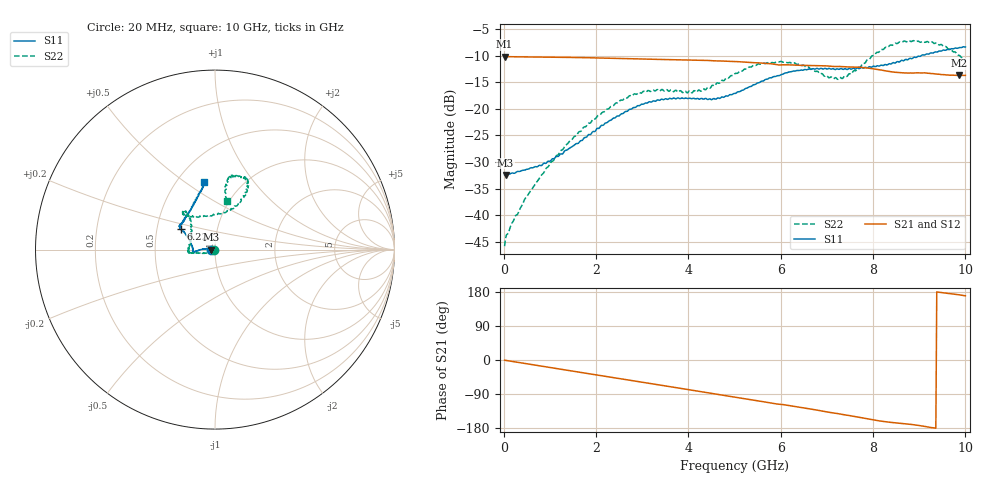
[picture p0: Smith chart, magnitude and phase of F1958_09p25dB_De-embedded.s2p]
! Integrated Device Technology
! Corporate Headquarters
! 6024 Silver Creek Valley Road
! San Jose, CA 95138  USA
! Phone:  1-408-284-8200
! Toll Free:  1-800-223-1366
! Webpage:  http://www.idt.com/
! Timing and RF Division
! 515 Groton Road, Suite 102
! Westford, MA 01886-6024
! Device:  F1958
! Description: 7-bit 0.25 dB Digital Step Attenuator
! Frequency:  0.001 -  6.000 GHz
! Package:  4x4 mm Thin QFN Plastic Package: 24 pin
! Ports:  2 RF, 12 DC
!  Pin  1  = D0
!  Pin  2  = VDD
!  Pin  3  = VMODE
!  Pin  4  = GND
!  Pin  5  = RF1  =  Port 1
!  Pin  6  = GND
!  Pin  7  = GND
!  Pin  8  = GND
!  Pin  9  = GND
!  Pin 10  = GND
!  Pin 11  = GND
!  Pin 12  = GND
!  Pin 13  = GND
!  Pin 14  = RF2  =  Port 2
!  Pin 15  = GND
!  Pin 16  = LE
!  Pin 17  = CLK
!  Pin 18  = DATA
!  Pin 19  = D6
!  Pin 20  = D5
!  Pin 21  = D4
!  Pin 22  = D3
!  Pin 23  = D2
!  Pin 24  = D1
! State:  37
! Atten State:  9.25 dB
! Voltage:  +3.30 Volts
! Current:  0.258 mA
! Data:  The device was measured on a F1958 evaluation board which has
!  individual transmission lines to the RF pins.  Data was collected
!  using a calibrated network analyzer.  The evaluation board was
!  de-embedded using Automatic Fixture Removal (AFR).
!  The reference plane is the edge of the package pin.
! Misc:
!  Action Tracker AT0419
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# GHz S dB R 50
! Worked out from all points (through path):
!   500 points, 20 MHz to 10 GHz, reference 50 ohm
!   highest |S21| = -10.19 dB at 20 MHz (marker M1); lowest = -13.7 dB at 9.86 GHz (marker M2)
!   group delay of S21, straight-line fit = 53.7 ps
!   lowest |S11| = -32.4 dB at 40 MHz (marker M3), VSWR 1.05, Z = 47.7 - j0.0687 ohm
!   |S11| at or under -10 dB: start of sweep to 9.048 GHz
!   |S22| runs from -45.8 to -7.2 dB; largest |S21 - S12| = 0.00084
!   S11 on the Smith chart (normalised r, x): 20 MHz: 0.95, -0.00; 6.22 GHz: 0.66, +0.16; 10 GHz: 0.67, +0.59
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0.02  -32.40 -178.2  -10.19 -0.5  -10.19 -0.5  -45.77 -157.7
0.04  -32.43 -178.3  -10.20 -0.9  -10.20 -0.9  -44.31 -151.7
0.22  -32.09 177.9  -10.23 -4.5  -10.23 -4.5  -40.86 -145.9
0.68  -30.84 173.9  -10.27 -13.5  -10.27 -13.4  -34.19 -144.1
1.16  -28.93 175.6  -10.31 -22.9  -10.31 -22.9  -28.71 -150.3
1.7  -25.92 176.7  -10.40 -33.3  -10.39 -33.3  -23.88 -162.4
2.58  -20.90 -176.9  -10.56 -50.5  -10.55 -50.5  -18.35 -171.0
3.36  -18.38 -171.8  -10.73 -65.7  -10.73 -65.8  -16.58 -175.4
4.22  -18.13 -175.0  -10.88 -82.4  -10.89 -82.5  -16.48 156.2
4.64  -17.95 175.6  -11.01 -90.6  -11.02 -90.7  -15.13 140.2
5.02  -17.10 164.5  -11.12 -98.2  -11.14 -98.2  -13.34 130.1
5.56  -14.93 153.1  -11.40 -108.8  -11.41 -108.8  -11.64 127.6
6.22  -13.05 148.9  -11.76 -121.2  -11.78 -121.1  -11.37 132.2
6.68  -12.51 146.5  -11.87 -130.0  -11.89 -129.9  -12.54 126.6
7.08  -12.53 143.4  -11.99 -138.7  -12.00 -138.6  -14.04 108.1
7.32  -12.45 141.4  -12.08 -143.3  -12.09 -143.2  -14.29 90.8
7.9  -12.20 129.8  -12.36 -155.7  -12.36 -155.8  -10.70 64.0
8.34  -11.57 120.3  -12.97 -164.0  -12.97 -164.1  -8.31 61.5
8.76  -10.75 111.8  -13.28 -169.2  -13.29 -169.2  -7.22 66.3
9.26  -9.49 104.3  -13.38 -178.2  -13.38 -178.3  -7.45 76.3
9.86  -8.54 99.4  -13.74 172.1  -13.77 172.2  -9.96 78.6
10  -8.40 99.4  -13.71 169.4  -13.75 169.5  -11.08 76.2
